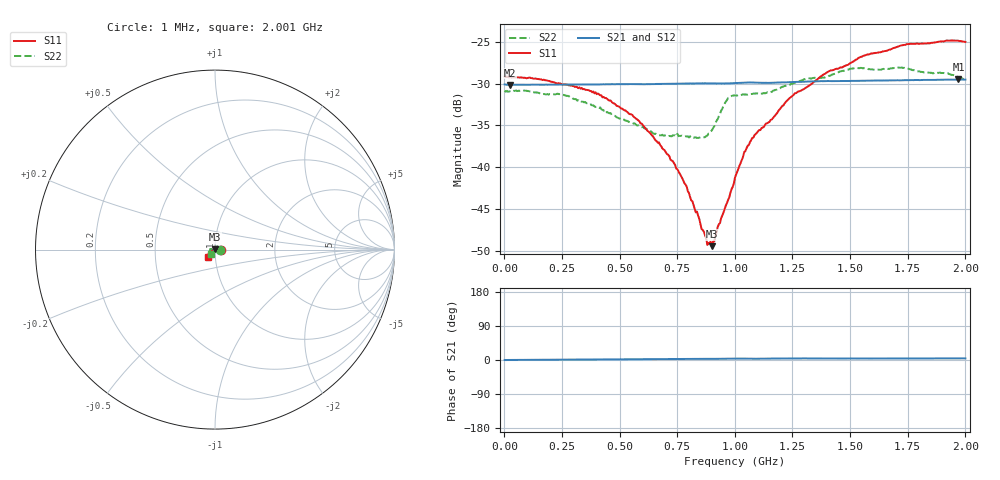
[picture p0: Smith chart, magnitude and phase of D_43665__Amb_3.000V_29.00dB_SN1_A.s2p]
! device id: 43665_
! dir: \\malibu\benchdata\1_engineers\tn_data\43665_75ohm\new\sparar\43665_\amb\3p000v\29p00db
! Serial: 1
! Insertion: A
! Temp: Amb
! VDD: 3.000V
! Attenuation Step: 29.00dB
! IDD: 1.450460e+00mA
! FILE NAME
! DATE 03-27-2009 08:40:30
! CORRECTED  DATA
#  Hz  S  RI  R  75
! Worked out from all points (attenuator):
!   401 points, 1 MHz to 2.001 GHz, reference 75 ohm
!   highest |S21| = -29.51 dB at 1.971 GHz (marker M1); lowest = -30.2 dB at 26 MHz (marker M2)
!   lowest |S11| = -49.4 dB at 901 MHz (marker M3), VSWR 1.01, Z = 74.7 + j0.378 ohm
!   |S11| at or under -10 dB: start of sweep to end of sweep
!   |S22| runs from -36.5 to -28.1 dB; largest |S21 - S12| = 0.00027
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1000000  0.0349 -0.00011  0.0313 0.000107  0.0311 -7.52e-05  0.0287 -0.000153
2.6e7  0.0346 0.000274  0.0311 5.92e-05  0.0311 7.05e-05  0.0285 0.00113
2.41e8  0.0314 0.00421  0.0312 0.000577  0.0312 0.000586  0.0247 0.0117
3.36e8  0.0293 0.00552  0.0312 0.000756  0.0312 0.000795  0.0196 0.0149
4.11e8  0.0264 0.00691  0.0312 0.000985  0.0313 0.001  0.0155 0.0164
5.56e8  0.0192 0.0071  0.0314 0.00114  0.0314 0.00121  0.00661 0.0172
6.71e8  0.0125 0.00648  0.0314 0.00149  0.0314 0.00153  -0.000801 0.0155
7.61e8  0.00738 0.00545  0.0315 0.0016  0.0316 0.0017  -0.00694 0.0138
7.96e8  0.00513 0.00508  0.0316 0.00163  0.0316 0.0017  -0.00949 0.012
8.76e8  -0.000332 0.00376  0.0317 0.00171  0.0317 0.00178  -0.0141 0.00624
9.01e8  -0.00224 0.00253  0.0317 0.00169  0.0317 0.00178  -0.0161 0.00413
9.61e8  -0.00583 0.000894  0.0317 0.00188  0.0317 0.00201  -0.0245 0.00305
1.001e9  -0.00867 0.00037  0.0318 0.00203  0.0318 0.00214  -0.0265 0.00433
1.046e9  -0.0124 -0.000848  0.032 0.00203  0.032 0.00212  -0.0271 0.00229
1.096e9  -0.0157 -0.0033  0.032 0.00187  0.032 0.00199  -0.0276 -0.000155
1.236e9  -0.0242 -0.0088  0.0321 0.0023  0.0322 0.0024  -0.03 -0.00819
1.336e9  -0.0285 -0.0137  0.0325 0.00238  0.0326 0.00249  -0.0314 -0.0131
1.546e9  -0.038 -0.0253  0.0328 0.00228  0.0329 0.00241  -0.0317 -0.0231
1.671e9  -0.0397 -0.0311  0.033 0.0023  0.0331 0.00243  -0.0297 -0.0249
1.756e9  -0.0404 -0.0365  0.0331 0.0023  0.0332 0.0024  -0.0274 -0.0274
1.971e9  -0.0382 -0.0423  0.0334 0.00252  0.0334 0.00254  -0.0222 -0.0264
2.001e9  -0.0372 -0.042  0.0333 0.00253  0.0334 0.00255  -0.021 -0.0254
